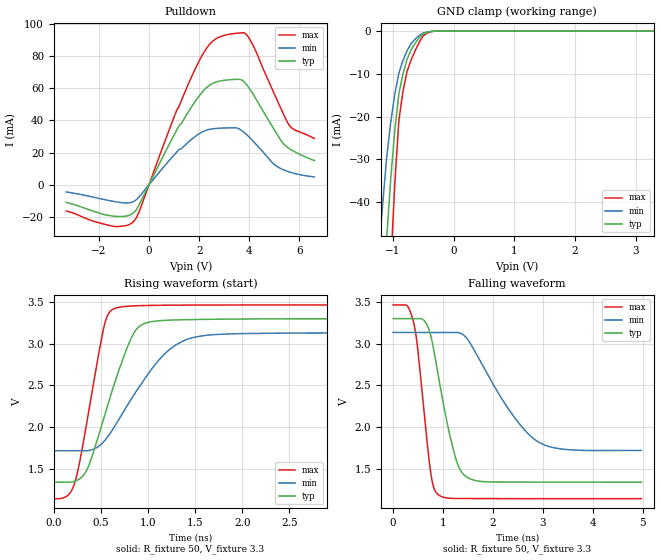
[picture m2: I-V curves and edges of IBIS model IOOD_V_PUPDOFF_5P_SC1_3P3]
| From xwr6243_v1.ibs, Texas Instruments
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|   Model Cell IOOD_V_PUPDOFF_5P_SC1_3P3
|IOOD_V_PUPDOFF_5P_SC1_3P3
[Model]   IOOD_V_PUPDOFF_5P_SC1_3P3
Model_type   I/O_open_drain
Polarity   Non-Inverting
Enable   Active-Low
Vinl =  0.8V
Vinh =  2V
Cref =  15pF
Rref =  100.0000M
Vref =  0V
Vmeas =  1.65
|   typ   min   max
C_comp   2.059994p   1.862014p   2.067327p
[Model Spec]
Vinl   0.8V   0.8V   0.8V
Vinh   2V   2V   2V
[Temperature Range]   25   125   -40
[Voltage Range]   3.3   3.135   3.465
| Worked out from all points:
|   slope of the pulldown table from 0 to 0.495 V, typ, clamps not added: 31.8 ohm
|   GND clamp passes 1 mA (typ) near -0.53 V on its own axis
|   rising waveform, R_fixture 50, V_fixture 3.3: 20-80 % time 334ps typ, 511ps min, 217ps max; typ from 1.34 V to 3.3 V
|   falling waveform, R_fixture 50, V_fixture 3.3: 20-80 % time 385ps typ, 889ps min, 239ps max; typ from 3.3 V to 1.34 V
| Where Nom  PVT is Nominal Process, 3.3V, 25C
|   Fast PVT is Strong Process,  3.465V, -40C
|   Slow PVT is Weak Process,   3.135V, 125C
[Pulldown]
|   voltage   I(typ)   I(min)   I(max)
-3.3V     -10.93mA   -4.474mA   -16.27mA
-1.4V     -19.53mA   -10.38mA   -25.83mA
-600mV    -17.23mA   -10.34mA   -22.61mA
1.2V      36.72mA    21.93mA    48.77mA
1.9V      53.02mA    30.66mA    73.76mA
2.4V      61.61mA    34.34mA    86.89mA
3V        64.86mA    35.24mA    92.76mA
3.6V      65.51mA    34.65mA    94.24mA
3.9V      62.01mA    31.1mA     93.16mA
5V        34.1mA     12.57mA    56.41mA
5.6V      22.42mA    7.958mA    36.79mA
6.6V      14.97mA    4.886mA    28.74mA
[GND_clamp]
|   voltage   I(typ)   I(min)   I(max)
-3.3V     -787.2mA   -627.7mA   -1.235A
-1.233V   -85.66mA   -52.14mA   -138.8mA
-1.167V   -66.47mA   -40.37mA   -107.7mA
-1.1V     -48.25mA   -29.37mA   -77.98mA
-1.033V   -34.27mA   -21.19mA   -54.56mA
-966.7mV  -23.06mA   -14.66mA   -35.5mA
-900mV    -14.61mA   -9.789mA   -20.83mA
-833.3mV  -10.05mA   -6.934mA   -14.15mA
-700mV    -4.416mA   -2.931mA   -6.81mA
-500mV    -621.6uA   -443.6uA   -1.094mA
-300mV    -17.13uA   -24.35uA   -23.51uA
3.3V      4.589uA    5.188uA    6.318uA
[Ramp]
| variable   typ   min   max
dV/dt_f  1.1805738/0.38563216n 0.85640964/0.89611487n  1.3985723/0.23982487n
dV/dt_r  1.1742367/0.46733695n 0.86227327/1.0179189n  1.4069723/0.25275808n
R_load = 50
[Rising Waveform]
R_fixture = 50
V_fixture = 3.3
V_fixture_min = 3.135
V_fixture_max = 3.465
|   time   V(typ)   V(min)   V(max)
0s        1.337V     1.714V     1.139V
145.7ps   1.337V     1.714V     1.176V
223.8ps   1.348V     1.714V     1.335V
357.9ps   1.502V     1.715V     2.102V
531ps     2.107V     1.824V     3.197V
639.5ps   2.506V     1.995V     3.42V
907.4ps   3.206V     2.483V     3.456V
1.198ns   3.281V     2.899V     3.461V
1.485ns   3.29V      3.074V     3.463V
4.974ns   3.3V       3.132V     3.465V
[Falling Waveform]
R_fixture = 50
V_fixture = 3.3
V_fixture_min = 3.135
V_fixture_max = 3.465
|   time   V(typ)   V(min)   V(max)
0s        3.3V       3.134V     3.464V
276.8ps   3.3V       3.134V     3.457V
412.9ps   3.3V       3.134V     3.247V
752.2ps   3.102V     3.134V     1.455V
907.9ps   2.605V     3.134V     1.184V
1.248ns   1.634V     3.134V     1.14V
1.512ns   1.385V     3.036V     1.138V
2.313ns   1.338V     2.213V     1.138V
2.894ns   1.337V     1.824V     1.138V
4.974ns   1.336V     1.717V     1.138V
